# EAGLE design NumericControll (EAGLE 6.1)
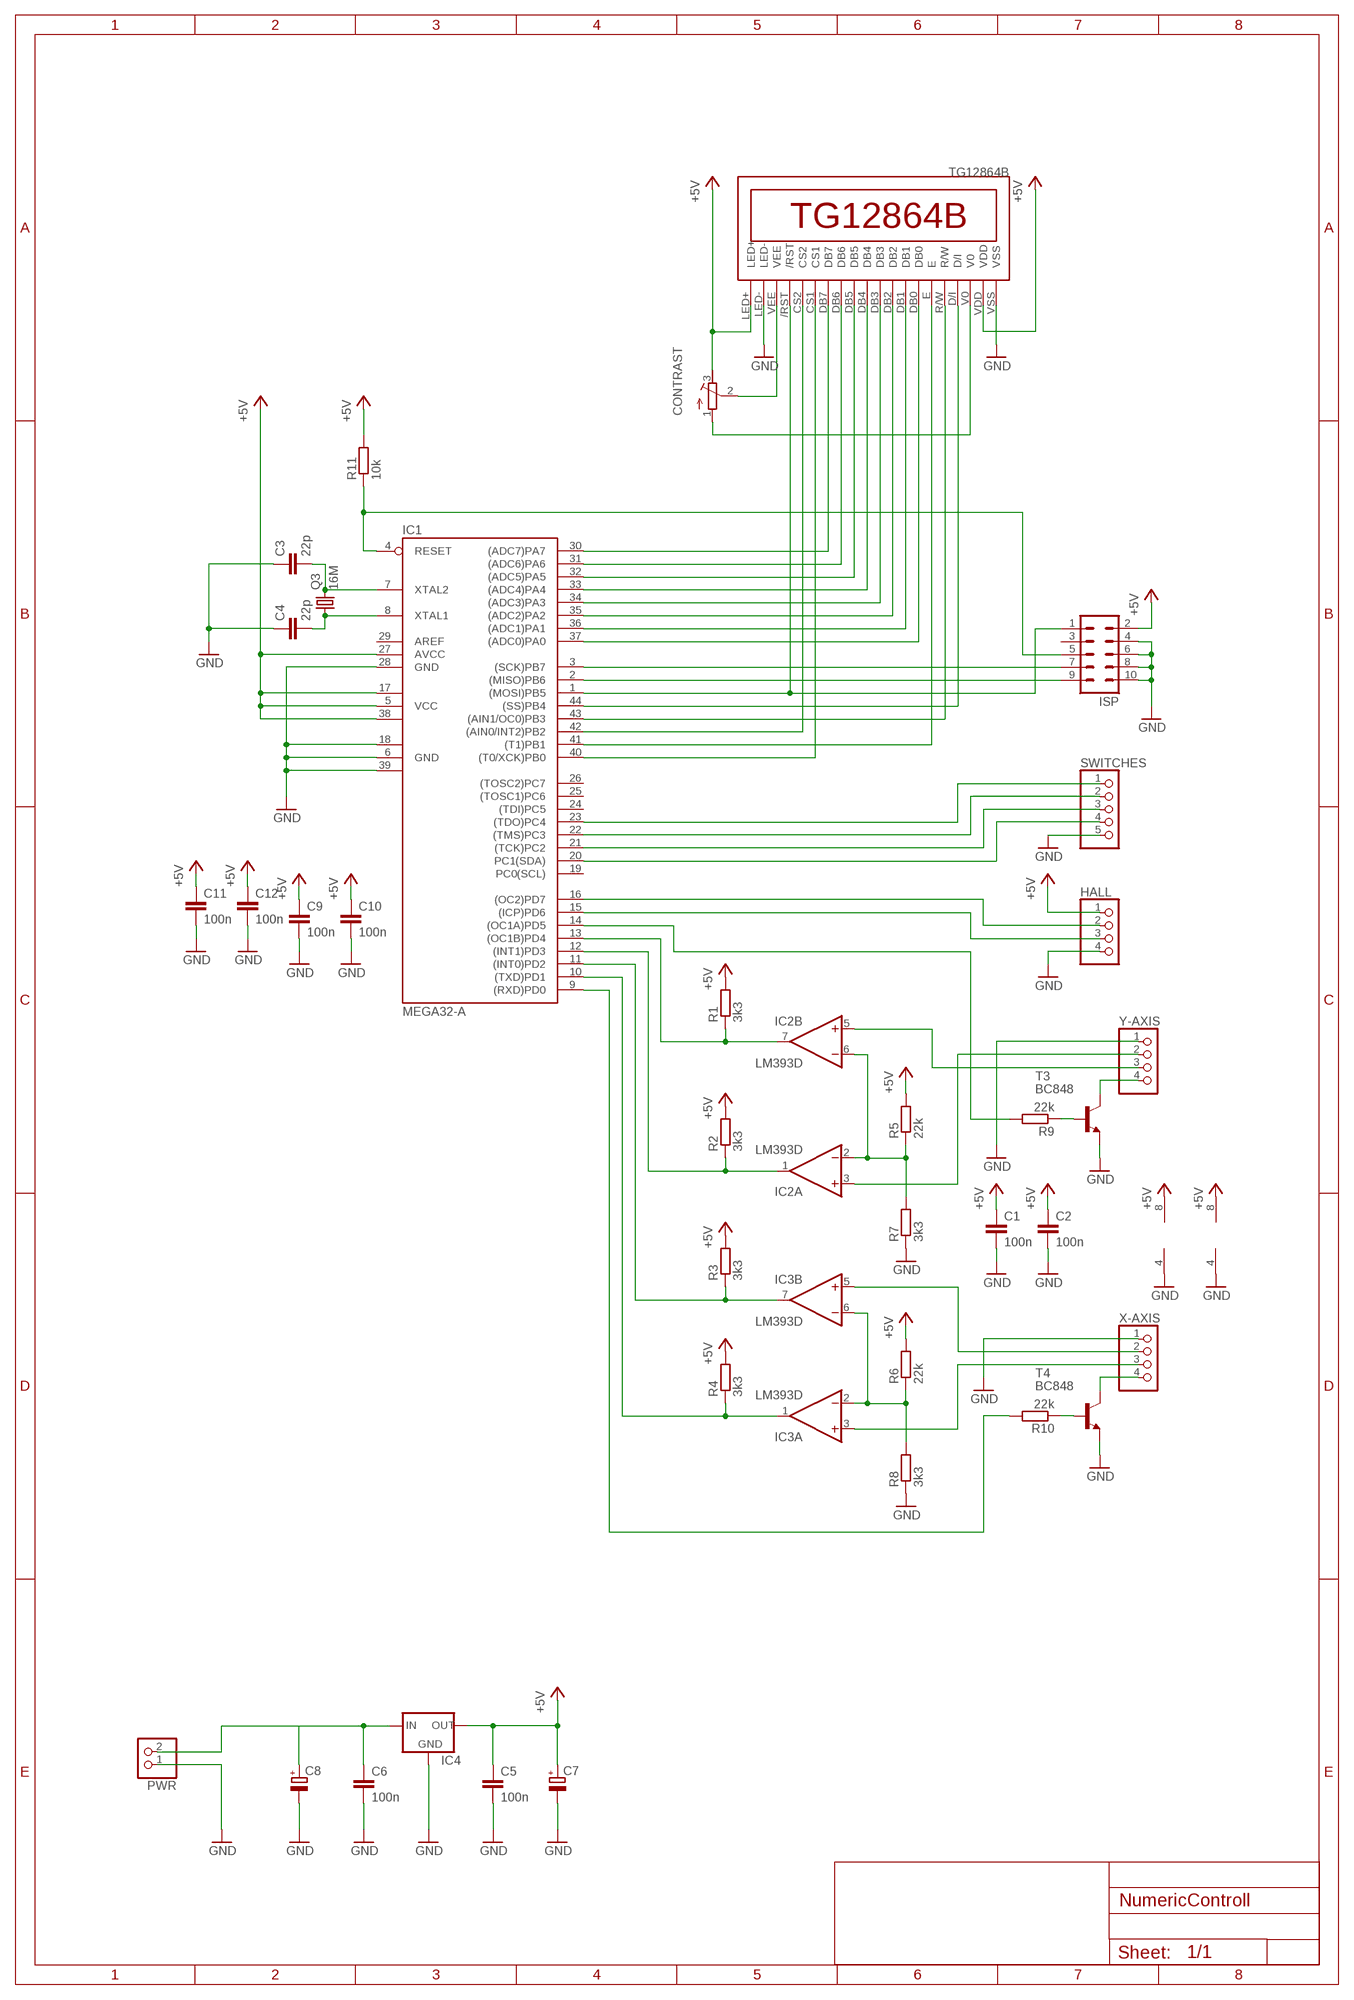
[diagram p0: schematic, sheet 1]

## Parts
C1  100n  C-EUC0805  [C0805]
C2  100n  C-EUC0805  [C0805]
C3  22p  C-EUC0805  [C0805]
C4  22p  C-EUC0805  [C0805]
C5  100n  C-EUC0805  [C0805]
C6  100n  C-EUC0805  [C0805]
C7  CPOL-EU153CLV-0505  [153CLV-0505]
C8  CPOL-EU153CLV-0505  [153CLV-0505]
C9  100n  C-EUC0805  [C0805]
C10  100n  C-EUC0805  [C0805]
C11  100n  C-EUC0805  [C0805]
C12  100n  C-EUC0805  [C0805]
CONTRAST  R-TRIMM3296X  [RTRIM3296X]
HALL  PINHD-1X4  [1X04]
IC1  MEGA32-A  [TQFP44]
IC2  LM393D  [SO08]
IC3  LM393D  [SO08]
IC4  78XXL  [78XXL]
ISP  ML10L  [ML10L]
PWR  PINHD-1X2  [1X02]
Q3  16M  CRYSTALHC49S  [HC49/S]
R1  3k3  R-EU_M0805  [M0805]
R2  3k3  R-EU_M0805  [M0805]
R3  3k3  R-EU_M0805  [M0805]
R4  3k3  R-EU_M0805  [M0805]
R5  22k  R-EU_M0805  [M0805]
R6  22k  R-EU_M0805  [M0805]
R7  3k3  R-EU_M0805  [M0805]
R8  3k3  R-EU_M0805  [M0805]
R9  22k  R-EU_M0805  [M0805]
R10  22k  R-EU_M0805  [M0805]
R11  10k  R-EU_M0805  [M0805]
SWITCHES  PINHD-1X5/90  [1X05/90]
T3  BC848  [SOT23]
T4  BC848  [SOT23]
U$1  TG12864B  [TG12864B]
X-AXIS  PINHD-1X4  [1X04]
Y-AXIS  PINHD-1X4  [1X04]

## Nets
+5V: C1.1 C2.1 C5.1 C7.+ C9.1 C10.1 C11.1 C12.1 CONTRAST.3(E) HALL.1 IC1.5(VCC) IC1.17(VCC1) IC1.27(AVCC) IC1.38(VCC2) IC2.8(P:V+) IC3.8(P:V+) IC4.OUT ISP.2 R1.2 R2.2 R3.2 R4.2 R5.2 R6.2 R11.2 U$1.LED+ U$1.VDD
GND: C1.2 C2.2 C3.1 C4.1 C5.2 C6.2 C7.- C8.- C9.2 C10.2 C11.2 C12.2 HALL.4 IC1.6(GND) IC1.18(GND1) IC1.28(GND) IC1.39(GND2) IC2.4(P:V-) IC3.4(P:V-) IC4.GND ISP.4 ISP.6 ISP.8 ISP.10 PWR.1 R7.1 R8.1 SWITCHES.5 T3.2(E) T4.2(E) U$1.LED- U$1.VSS X-AXIS.1 Y-AXIS.1
N$1: IC1.30((ADC7)PA7) U$1.DB7
N$2: IC1.31((ADC6)PA6) U$1.DB6
N$3: IC1.32((ADC5)PA5) U$1.DB5
N$4: IC1.33((ADC4)PA4) U$1.DB4
N$5: IC1.34((ADC3)PA3) U$1.DB3
N$6: IC1.35((ADC2)PA2) U$1.DB2
N$7: IC1.36((ADC1)PA1) U$1.DB1
N$8: IC1.37((ADC0)PA0) U$1.DB0
N$9: IC1.12((INT1)PD3) IC2.1(A:OUT) R2.1
N$10: IC1.13((OC1B)PD4) IC2.7(B:OUT) R1.1
N$11: IC1.11((INT0)PD2) IC3.7(B:OUT) R3.1
N$12: IC1.14((OC1A)PD5) R9.2
N$13: IC1.10((TXD)PD1) IC3.1(A:OUT) R4.1
N$14: IC3.2(A:-IN) IC3.6(B:-IN) R6.1 R8.2
N$15: IC2.2(A:-IN) IC2.6(B:-IN) R5.1 R7.2
N$16: IC2.3(A:+IN) Y-AXIS.2
N$17: IC2.5(B:+IN) Y-AXIS.3
N$18: IC3.3(A:+IN) X-AXIS.3
N$19: IC3.5(B:+IN) X-AXIS.2
N$20: IC1.9((RXD)PD0) R10.2
N$21: T3.3(C) Y-AXIS.4
N$22: R9.1 T3.1(B)
N$23: IC1.3((SCK)PB7) ISP.7
N$24: IC1.2((MISO)PB6) ISP.9
N$25: IC1.1((MOSI)PB5) ISP.1 U$1./RST
N$26: T4.3(C) X-AXIS.4
N$27: R10.1 T4.1(B)
N$28: IC1.4(RESET) ISP.5 R11.1
N$29: C3.2 IC1.7(XTAL2) Q3.2
N$30: C4.2 IC1.8(XTAL1) Q3.1
N$31: IC1.22((TMS)PC3) SWITCHES.2
N$32: IC1.21((TCK)PC2) SWITCHES.3
N$33: IC1.23((TDO)PC4) SWITCHES.1
N$34: IC1.20(PC1(SDA)) SWITCHES.4
N$35: HALL.2 IC1.16((OC2)PD7)
N$36: HALL.3 IC1.15((ICP)PD6)
N$37: CONTRAST.2(S) U$1.VEE
N$38: CONTRAST.1(A) U$1.V0
N$40: IC1.44((SS)PB4) U$1.D/I
N$41: IC1.43((AIN1/OC0)PB3) U$1.R/W
N$42: IC1.41((T1)PB1) U$1.E
N$43: IC1.40((T0/XCK)PB0) U$1.CS1
N$44: IC1.42((AIN0/INT2)PB2) U$1.CS2
N$46: C6.1 C8.+ IC4.IN PWR.2
Unconnected: IC1.19(PC0(SCL)) IC1.24((TDI)PC5) IC1.25((TOSC1)PC6) IC1.26((TOSC2)PC7) IC1.29(AREF) ISP.3

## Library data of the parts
C1-C6 C9-C12 = rcl:C-EU: CAPACITOR, European symbol
C7 C8 = rcl:CPOL-EU: POLARIZED CAPACITOR, European symbol
CONTRAST = rcl:R-TRIMM: Trimm resistor
HALL X-AXIS Y-AXIS = pinhead:PINHD-1X4: PIN HEADER
IC1 = atmel:MEGA32: MICROCONTROLLER 32 Kbytes FLASH 2 Kbytes SRAM 1 Kbytes EEPROM USART 8-channel 10 bit ADC Source: www.atmel.com .. doc2503.pdf; MPN: ATMEGA32-16AU; OC_FARNELL: 9171274; OC_NEWARK: 69K6677
IC2 IC3 = linear:LM393: COMPARATOR
IC4 = v-reg:78XXL: VOLTAGE REGULATOR
ISP = con-harting-ml:ML10: HARTING; OC_FARNELL: unknown; OC_NEWARK: unknown
PWR = pinhead:PINHD-1X2: PIN HEADER
Q3 = crystal:CRYSTAL: CRYSTAL; OC_FARNELL: 1667008; OC_NEWARK: unknown
R1-R11 = rcl:R-EU_: RESISTOR, European symbol
SWITCHES = pinhead:PINHD-1X5: PIN HEADER
T3 T4 = transistor:BC848: NPN TRANSISTOR
U$1 = TG12864B:TG12864B

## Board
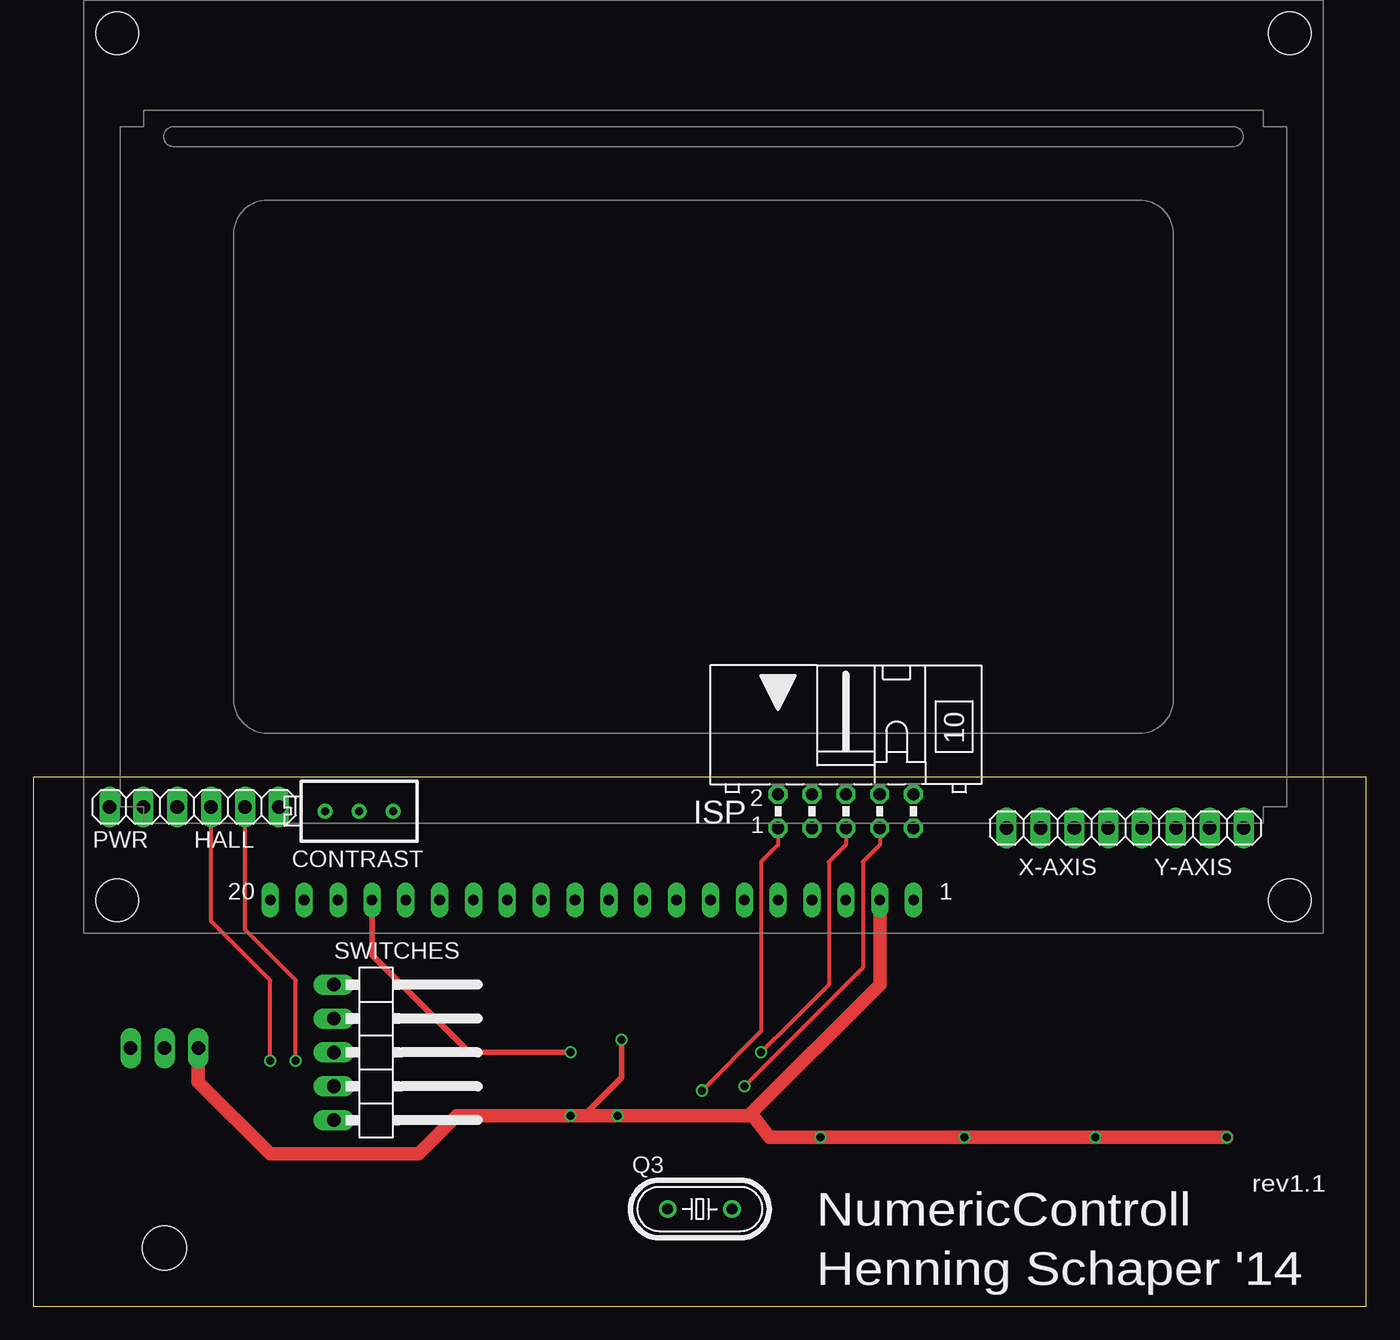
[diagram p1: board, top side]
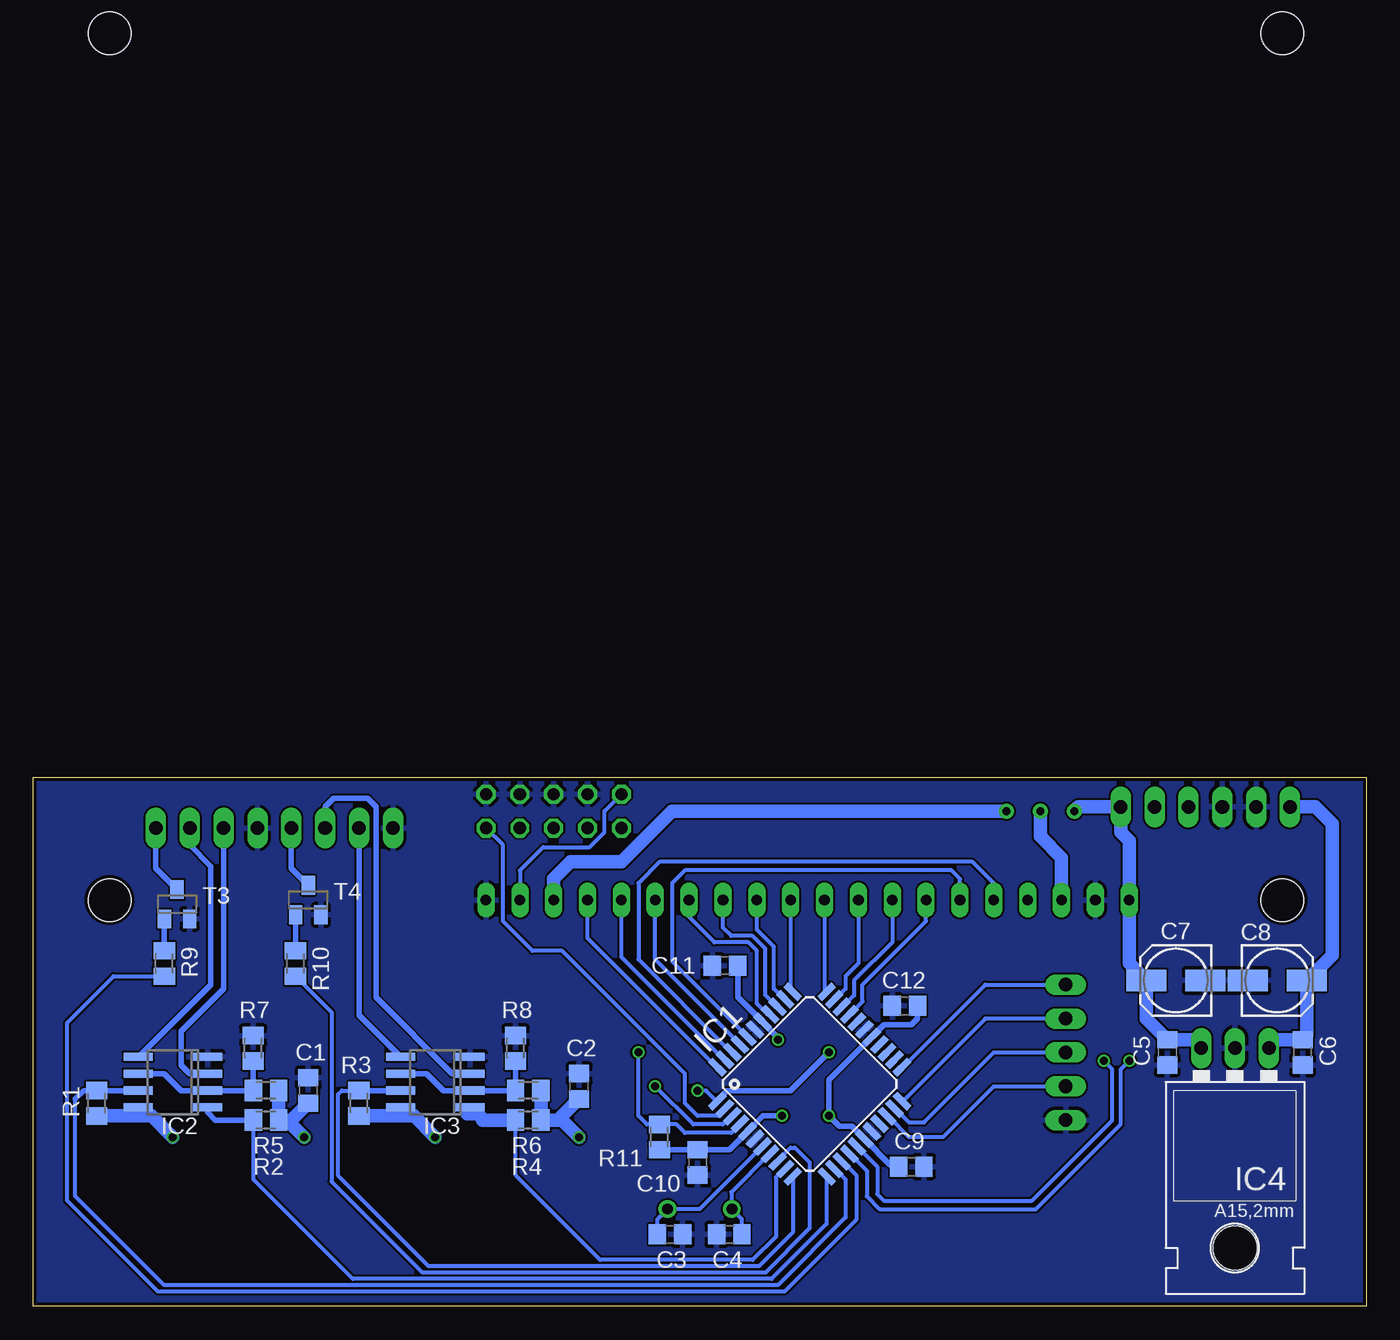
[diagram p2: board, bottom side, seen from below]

Size 100 x 39.67 mm. Coordinates in mm from the lower left corner, seen from the top.
Outline: 0,0 100,0 100,39.67 0,39.67 0,0
Copper layers (1*16): Top 0.035mm / dielectric 1.5mm / Bottom 0.035mm
Design rules: minimum track width 6mil, minimum drill 12mil, track to track 6mil, track to pad 6mil, pad to pad 6mil, via to via 6mil, smd to smd 0mil, copper to edge 10mil, drill to drill 10mil, minimum pad ring 10mil, minimum via ring 6mil, stop-mask expansion 2mil, vias tented up to drill 100mil, thermal gap 10mil

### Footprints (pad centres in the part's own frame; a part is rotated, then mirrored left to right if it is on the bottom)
C0805 = smd 1.3 x 1.5: 1 -0.95,0; 2 0.95,0
153CLV-0505 = smd 3 x 1.6: + 2.2,0; - -2.2,0
RTRIM3296X = drill 0.61: 1 0,-2.54; 2 0,0; 3 0,2.54
1X04 = drill 1.016 long: 1 -3.81,0; 2 -1.27,0; 3 1.27,0; 4 3.81,0
TQFP44 = smd 1.5 x 0.5: 1 -5.8,4; 2 -5.8,3.2; 3 -5.8,2.4; 4 -5.8,1.6; 5 -5.8,0.8; 6 -5.8,0; 7 -5.8,-0.8; 8 -5.8,-1.6; 9 -5.8,-2.4; 10 -5.8,-3.2; 11 -5.8,-4; 23 5.8,-4; 24 5.8,-3.2; 25 5.8,-2.4; 26 5.8,-1.6; 27 5.8,-0.8; 28 5.8,0; 29 5.8,0.8; 30 5.8,1.6; 31 5.8,2.4; 32 5.8,3.2; 33 5.8,4 | smd 0.5 x 1.5: 12 -4,-5.8; 13 -3.2,-5.8; 14 -2.4,-5.8; 15 -1.6,-5.8; 16 -0.8,-5.8; 17 0,-5.8; 18 0.8,-5.8; 19 1.6,-5.8; 20 2.4,-5.8; 21 3.2,-5.8; 22 4,-5.8; 34 4,5.8; 35 3.2,5.8; 36 2.4,5.8; 37 1.6,5.8; 38 0.8,5.8; 39 0,5.8; 40 -0.8,5.8; 41 -1.6,5.8; 42 -2.4,5.8; 43 -3.2,5.8; 44 -4,5.8
SO08 = smd 0.6 x 2.2: 1 -1.905,-2.6; 2 -0.635,-2.6; 3 0.635,-2.6; 4 1.905,-2.6; 5 1.905,2.6; 6 0.635,2.6; 7 -0.635,2.6; 8 -1.905,2.6
78XXL = drill 1.016 long: GND 0,-3.81; IN -2.54,-3.81; OUT 2.54,-3.81 | hole 3.302: 0,11.176
ML10L = drill 0.914 octagon: 1 -5.08,-1.27; 2 -5.08,1.27; 3 -2.54,-1.27; 4 -2.54,1.27; 5 0,-1.27; 6 0,1.27; 7 2.54,-1.27; 8 2.54,1.27; 9 5.08,-1.27; 10 5.08,1.27
1X02 = drill 1.016 long: 1 -1.27,0; 2 1.27,0
HC49/S = drill 0.813: 1 -2.413,0; 2 2.413,0
M0805 = smd 1.3 x 1.6: 1 -0.95,0; 2 0.95,0
1X05/90 = drill 1.016 long: 1 -5.08,-3.81; 2 -2.54,-3.81; 3 0,-3.81; 4 2.54,-3.81; 5 5.08,-3.81
SOT23 = smd 1 x 1.4: 1 -0.95,-1.1; 2 0.95,-1.1; 3 0,1.1
TG12864B = drill 0.8 long: /RST 7.62,0; CS1 12.7,0; CS2 10.16,0; D/I 40.64,0; DB0 33.02,0; DB1 30.48,0; DB2 27.94,0; DB3 25.4,0; DB4 22.86,0; DB5 20.32,0; DB6 17.78,0; DB7 15.24,0; E 35.56,0; LED+ 0,0; LED- 2.54,0; R/W 38.1,0; V0 43.18,0; VDD 45.72,0; VEE 5.08,0; VSS 48.26,0 | hole 3.2: -11.5,0; 76.5,0; -11.5,65; 76.5,65

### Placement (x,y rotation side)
C1  79.38,16.19 90 bottom
C2  59.05,16.51 90 bottom
C3  52.23,5.4 180 bottom
C4  47.78,5.4 0 bottom
C5  14.92,19.05 270 bottom
C6  4.76,19.05 270 bottom
C7  14.29,24.45 180 bottom
C8  6.67,24.45 0 bottom
C9  34.13,10.48 0 bottom
C10  50.16,10.79 270 bottom
C11  48.1,25.56 180 bottom
C12  34.61,22.54 180 bottom
CONTRAST  24.45,37.15 90 top
HALL  14.61,37.46 180 top
IC1  41.75,16.67 45 bottom
IC2  89.53,16.83 90 bottom
IC3  69.85,16.83 90 bottom
IC4  9.84,15.56 180 bottom
ISP  60.96,37.15 0 top
PWR  6.99,37.46 180 top
Q3  50.01,7.3 0 top
R1  95.25,15.24 270 bottom
R2  82.55,13.97 0 bottom
R3  75.56,15.24 270 bottom
R4  62.87,13.97 0 bottom
R5  82.55,16.19 0 bottom
R6  62.87,16.19 0 bottom
R7  83.5,19.37 270 bottom
R8  63.82,19.37 270 bottom
R9  90.17,25.72 270 bottom
R10  80.33,25.72 270 bottom
R11  53.02,12.7 270 bottom
SWITCHES  26.35,19.05 270 top
T3  89.22,30.16 0 bottom
T4  79.38,30.48 0 bottom
U$1  17.78,30.48 0 top
X-AXIS  76.83,35.88 0 top
Y-AXIS  87,35.88 0 top

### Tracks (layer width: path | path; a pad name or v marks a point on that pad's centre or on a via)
+5V  (via drill 0.6)
  Top 0.305: 44.61,14.45 44.45,14.29
  Top 0.406: v44.13,20 44.13,17.14 41.27,14.29
  Top 1.016: 53.66,14.29 63.5,24.13 U$1.VDD | 53.66,14.29 44.45,14.29 v43.81,14.29 41.27,14.29 v40.32,14.29 31.75,14.29 28.89,11.43 17.78,11.43 12.38,16.83 IC4.OUT | 53.66,14.29 53.98,14.29 55.24,12.7 v59.05,12.7 v69.85,12.7 v79.69,12.7 v89.53,12.7
  Bottom 0.254: C7.+ 16.51,24.45
  Bottom 0.305: 37.33,19.82 IC1.27 37.08,20.22 | ISP.2 57.15,37.15 57.15,35.56 58.26,34.45 61.75,34.45 63.5,32.7 U$1.VDD | C12.1 | IC1.17 | 35.72,10.64 35.24,10.64 C9.1 | IC1.5 46.42,13.11 | 47.78,11.75 C10.1 | R11.2 C10.1 | IC1.17
  Bottom 0.406: IC1.27 37.49,19.82 40.32,16.99 v40.32,14.29 39.53,13.49 38.58,13.49 IC1.17 35.72,10.64 | 93.03,14.29 92.71,14.29 92.14,14.86 IC2.8 93.03,14.03 | R1.2 | R3.2 73.08,14.29 | 73.08,14.29 IC3.8 | 73.34,14.03 73.08,14.29 | 37.08,20.22 36.2,21.11 34.13,21.11 33.66,21.59 C12.1 | 46.42,13.11 47.78,11.75 R11.2 | v44.13,20 44.13,20.16 45.29,21.32 IC1.38 45.31,21.34 47.15,23.18 C11.1 | IC1.5 46.4,13.13 45.24,14.29 v43.81,14.29
  Bottom 1.016: IC4.OUT 13.02,20 C5.1 16.49,21.56 C7.+ | CONTRAST.3 21.59,37.46 HALL.1 18.41,35.56 17.78,34.92 U$1.LED+ 17.78,25.72 16.51,24.45 | R5.2 R2.2 80.96,13.97 | R1.2 93.03,14.29 91.12,14.29 v89.53,12.7 | R6.2 R4.2 60.33,13.97 | 60.33,13.97 v59.05,12.7 | R3.2 71.44,14.29 v69.85,12.7 | 80.96,13.97 v79.69,12.7 | C1.1 80.64,13.97 80.96,13.97 | 60.33,13.97 60.33,14.29 C2.1
GND
  pour Bottom: -0.32,40 100.65,40 100.65,-0.64 -0.32,-0.32
N$1
  Bottom 0.305: 39.01,21.63 IC1.30 38.74,21.9 37.78,22.86 37.78,24.13 33.02,28.89 U$1.DB7
N$2
  Bottom 0.305: U$1.DB6 35.56,27.3 38.42,24.45 38.42,23.32 39.27,22.47 IC1.31
N$3
  Bottom 0.305: U$1.DB5 38.1,25.72 39.05,24.77 39.05,23.82 39.84,23.03 IC1.32
N$4
  Bottom 0.305: 40.64,23.38 IC1.33 40.64,23.76 U$1.DB4
N$5
  Bottom 0.305: U$1.DB3 43.18,23.75 IC1.34
N$6
  Bottom 0.305: IC1.35 43.67,23.03 44.45,23.81 44.45,26.99 45.72,28.26 U$1.DB2
N$7
  Bottom 0.305: IC1.36 44.22,22.47 45.09,23.34 45.09,26.83 46.04,27.78 47.62,27.78 48.26,28.42 U$1.DB1
N$8
  Bottom 0.305: U$1.DB0 50.8,29.21 48.9,27.3 46.35,27.3 45.72,26.67 45.72,22.7 44.92,21.9 IC1.37
N$9
  Bottom 0.305: R2.1 83.5,9.53 76.04,2.06 44.61,2.06 40.48,6.19 IC1.12
  Bottom 0.406: IC2.1 86.94,14.54 86.36,13.97 R2.1
N$10
  Bottom 0.305: 96.84,15.56 96.84,8.26 90.17,1.59 44.13,1.59 39.05,6.67 39.05,9.53 39.83,10.31 IC1.13
  Bottom 0.406: IC2.7 R1.1 96.2,16.19 96.84,15.56
N$11
  Bottom 0.305: R3.1 76.83,16.19 77.15,15.88 77.15,9.84 70.33,3.02 45.56,3.02 43.02,5.55 IC1.11
  Bottom 0.406: R3.1 IC3.7
N$12
  Bottom 0.305: R9.2 93.98,24.77 97.47,21.27 97.47,7.94 90.65,1.11 43.66,1.11 38.26,6.51 38.26,9.84 39.29,10.87 IC1.14
  Bottom 0.406: R9.2
N$13
  Bottom 0.305: R4.1 63.82,9.84 57.47,3.49 46.04,3.49 44.29,5.24 44.29,9.68 43.67,10.31 IC1.10
  Bottom 0.406: 67.47,14.45 67.47,14.7 IC3.1
  Bottom 1.016: R4.1 66.3,13.97 66.3,14.07 66.67,14.45 67.47,14.45
N$14
  Bottom 0.406: R8.2 R6.1 IC3.2 69.22,16.19 70.48,17.46 IC3.6
N$15
  Bottom 0.254: R5.1
  Bottom 0.406: R5.1 IC2.2 88.9,16.19 90.17,17.46 IC2.6 | R7.2 R5.1
N$16
  Bottom 0.406: Y-AXIS.2 85.72,23.81 88.9,20.64 88.9,18.1 88.27,17.46 IC2.3
N$17
  Bottom 0.406: IC2.5 92.08,18.73 86.68,24.13 86.68,33.02 88.27,34.61 Y-AXIS.3
N$18
  Bottom 0.406: IC3.3 68.58,17.46 74.3,23.18 74.3,37.46 74.93,38.1 77.47,38.1 78.11,37.46 X-AXIS.3
N$19
  Bottom 0.406: X-AXIS.2 75.56,21.85 IC3.5
N$20
  Bottom 0.254: R10.2
  Bottom 0.305: R10.2 77.63,22.07 77.63,9.37 70.8,2.54 45.09,2.54 41.75,5.87 41.75,10.79 42.86,11.91 43.18,11.91 44.16,10.93 IC1.9
N$21
  Bottom 0.406: Y-AXIS.4 90.81,32.85 T3.3
N$22
  Bottom 0.406: R9.1 T3.1
N$23  (via drill 0.6)
  Top 0.305: v53.34,16.51 62.23,25.4 62.23,33.34 63.5,34.61 ISP.7
  Bottom 0.305: v53.34,16.51 50.48,13.65 48.26,13.65 47.65,14.27 IC1.3
N$24
  Bottom 0.305: ISP.9 64.77,34.61 64.77,28.89 62.55,26.67 60.33,26.67 51.12,17.46 51.12,15.24 50.16,14.29 48.58,14.29 48.12,14.75 IC1.2
N$25  (via drill 0.6)
  Top 0.305: v50.16,16.19 54.61,20.64 54.61,33.34 55.88,34.61 ISP.1
  Top 0.406: v40.32,19.05 32.7,19.05 25.4,26.35 U$1./RST
  Bottom 0.305: 25.4,29.53 U$1./RST | IC1.1 48.73,15.4 49.53,16.19 v50.16,16.19
  Bottom 0.406: IC1.1 48.68,15.45 47.94,16.19 43.18,16.19 v40.32,19.05
N$26
  Bottom 0.406: X-AXIS.4 80.64,32.85 T4.3
N$27
  Bottom 0.406: R10.1 T4.1
N$28  (via drill 0.6)
  Top 0.305: v54.61,19.05 56.83,21.27 57.15,21.59 59.69,24.13 59.69,33.34 60.96,34.61 ISP.5
  Bottom 0.305: IC1.4 46.98,13.66 47.62,13.02 51.12,13.02 51.75,13.65 R11.1 | R11.1 53.97,13.65 54.61,14.29 v54.61,19.05
  Bottom 0.406: R11.1
N$29
  Bottom 0.305: IC1.7 45.31,12 50.01,7.3 Q3.2 53.02,6.7 53.02,6.67 53.18,6.51 C3.2
N$30
  Bottom 0.305: IC1.8 44.76,11.44 47.62,8.57 47.62,7.33 Q3.1 46.83,6.54 C4.2
N$31
  Bottom 0.305: SWITCHES.2 28.57,21.59 34.77,15.4 IC1.22
N$32
  Bottom 0.305: SWITCHES.3 27.94,19.05 33.18,13.81 34.29,13.81 35.31,14.83 IC1.21
N$33
  Bottom 0.305: 35.25,17.46 IC1.23 34.76,17.94 28.57,24.13 SWITCHES.1
N$34
  Bottom 0.305: SWITCHES.4 27.94,16.51 31.75,12.7 34.29,12.7 35.85,14.27 IC1.20
N$35  (via drill 0.6)
  Top 0.305: v19.68,18.41 19.68,24.45 15.88,28.26 HALL.2
  Bottom 0.305: v19.68,18.41 19.05,17.78 19.05,13.97 25.08,7.94 36.2,7.94 36.67,8.41 36.67,10.48 38.2,12 IC1.16
N$36  (via drill 0.6)
  Top 0.305: v17.78,18.41 17.78,24.45 13.34,28.89 HALL.3
  Bottom 0.305: v17.78,18.41 18.41,17.78 18.41,13.65 24.77,7.3 36.51,7.3 37.47,8.26 37.47,10.16 38.74,11.44 IC1.15
N$37
  Bottom 1.016: U$1.VEE 22.86,33.66 24.45,35.24 CONTRAST.2
N$38
  Bottom 1.016: CONTRAST.1 52.07,37.15 55.88,33.34 59.69,33.34 60.96,32.07 U$1.V0
N$40
  Bottom 0.305: U$1.D/I 58.42,27.62 48.74,17.94 IC1.44
N$41
  Bottom 0.305: U$1.R/W 55.88,26.19 48.19,18.51 IC1.43
N$42
  Bottom 0.305: U$1.E 53.34,26.04 46.98,19.68 IC1.41
N$43
  Bottom 0.305: U$1.CS1 30.48,32.07 31.11,32.7 51.12,32.7 52.07,31.75 52.07,25.88 46.42,20.22 IC1.40
N$44
  Bottom 0.305: U$1.CS2 27.94,31.75 29.53,33.34 53.02,33.34 54.61,31.75 54.61,26.04 47.91,19.33 IC1.42
N$46
  Bottom 0.254: C8.+ 4.45,24.45 | C6.1
  Bottom 1.016: PWR.2 3.81,37.46 2.54,36.2 2.54,26.35 4.45,24.45 4.45,20.32 C6.1 | C6.1 6.67,20 IC4.IN

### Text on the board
tNames: rev1.1 | NumericControll | Henning Schaper '14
